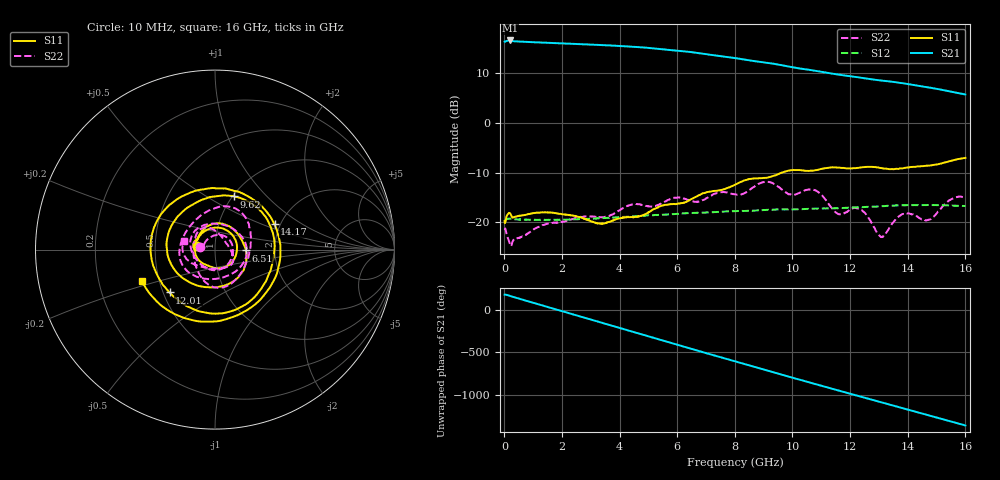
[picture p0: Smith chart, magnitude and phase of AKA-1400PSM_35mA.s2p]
!Keysight Technologies,P9375A,MY57211602,A.15.55.08
!Date: Tuesday, April 18, 2023 17:01:12
!Correction: S11(Cdelta 2-Port  )
!S21(Cdelta 2-Port  )
!S12(Cdelta 2-Port  )
!S22(Cdelta 2-Port  )
!S2P File: Measurements: S11, S21, S12, S22:
# Hz S  dB  R 50
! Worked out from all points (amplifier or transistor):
!   1600 points, 10 MHz to 16 GHz, reference 50 ohm
!   highest |S21| = 16.5 dB at 200 MHz (marker M1)
!   |S21| within 3 dB of that: start of sweep to 7.326 GHz
!   unconditionally stable (mu >= 1): start of sweep to end of sweep
!   at 2.67 GHz: K = 1.08, MAG = 15.8 dB, |S12| = -19.3 dB
!   at 8.01 GHz: K = 1.11, MAG = 13.3 dB, |S12| = -17.7 dB
!   at 16 GHz: K = 1.59, MAG = 6.7 dB, |S12| = -16.7 dB
!   S11 on the Smith chart (normalised r, x): 10 MHz: 0.82, +0.03; 6.51 GHz: 1.42, -0.01; 9.62 GHz: 1.02, +0.67; 12.01 GHz: 0.54, -0.29; 14.17 GHz: 1.87, +0.60; 16 GHz: 0.40, -0.18
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1e7  -19.73 168.6  16.25 175.7  -19.43 -3.5  -21.44 171.5
2e8  -18.15 158.5  16.48 159.4  -19.21 -17.4  -24.47 154.0
9.1e8  -18.26 90.0  16.16 88.6  -19.47 -76.4  -21.85 87.6
1.65e9  -18.03 20.4  15.96 15.6  -19.46 -137.6  -20.12 19.9
2.11e9  -18.39 -17.8  15.86 -29.6  -19.42 -175.5  -19.78 -23.9
2.68e9  -19.04 -63.2  15.72 -85.7  -19.32 137.2  -18.89 -71.0
3.27e9  -20.18 -105.2  15.59 -143.8  -19.14 88.4  -18.91 -115.2
3.73e9  -19.69 -134.9  15.46 170.7  -19.06 49.7  -18.45 -156.6
4.53e9  -18.88 160.3  15.18 91.8  -18.77 -17.1  -16.29 138.2
5.34e9  -16.97 96.1  14.80 11.7  -18.51 -85.9  -16.50 56.4
6e9  -16.24 37.6  14.44 -53.1  -18.27 -141.7  -15.01 -6.4
6.51e9  -15.26 -1.6  14.13 -103.6  -18.09 174.5  -15.70 -56.2
7.25e9  -13.73 -70.8  13.53 -176.1  -17.95 111.1  -14.35 -135.5
8.01e9  -12.40 -138.8  12.95 109.8  -17.71 45.5  -14.39 159.1
8.89e9  -11.14 133.8  12.17 25.4  -17.55 -29.6  -12.12 76.2
9.62e9  -10.04 70.3  11.53 -45.0  -17.42 -93.0  -13.37 22.6
1.067e10  -9.64 -23.4  10.52 -144.0  -17.25 177.2  -13.37 -82.5
1.201e10  -9.17 -136.7  9.31 89.8  -17.01 61.7  -17.37 139.1
1.334e10  -9.28 103.3  8.28 -34.6  -16.66 -53.5  -21.24 -0.4
1.417e10  -8.86 23.0  7.59 -112.7  -16.53 -126.6  -18.37 -50.6
1.497e10  -8.40 -58.6  6.81 172.6  -16.52 163.5  -18.43 -126.8
1.6e10  -7.06 -156.4  5.66 77.7  -16.70 74.1  -14.93 164.6
